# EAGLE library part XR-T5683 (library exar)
8 MBPS PCM LINE INTERFACE
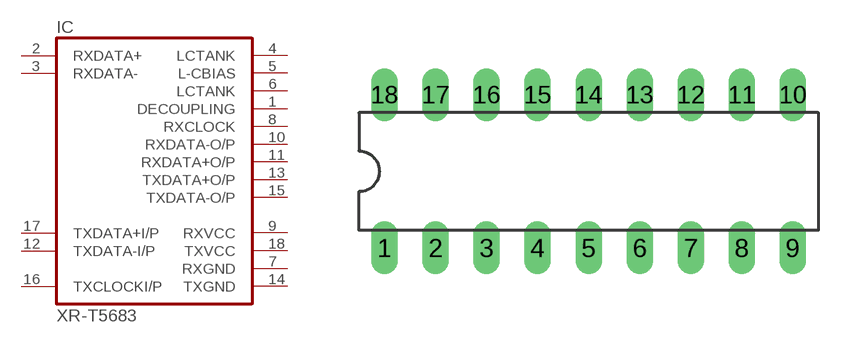
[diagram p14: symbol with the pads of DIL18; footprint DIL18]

Designator prefix IC

## XR-T5683 (OC_FARNELL: unknown; OC_NEWARK: unknown)  [DIL18]
1  DECOUPLING  out
2  RXDATA+  in
3  RXDATA-  in
4  LCTANK  out
5  L-CBIAS  out
6  LCTANK  out
7  RXGND  pwr
8  RXCLOCK  out
9  RXVCC  pwr
10  RXDATA-O/P  out
11  RXDATA+O/P  out
12  TXDATA-I/P  in
13  TXDATA+O/P  out
14  TXGND  pwr
15  TXDATA-O/P  out
16  TXCLOCKI/P  in
17  TXDATA+I/P  in
18  TXVCC  pwr

## Footprint DIL18 (pad centres in mm)
Dual In Line Package
drill 0.813 long: 1 -10.16,-3.81; 2 -7.62,-3.81; 3 -5.08,-3.81; 4 -2.54,-3.81; 5 0,-3.81; 6 2.54,-3.81; 7 5.08,-3.81; 8 7.62,-3.81; 9 10.16,-3.81; 10 10.16,3.81; 11 7.62,3.81; 12 5.08,3.81; 13 2.54,3.81; 14 0,3.81; 15 -2.54,3.81; 16 -5.08,3.81; 17 -7.62,3.81; 18 -10.16,3.81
